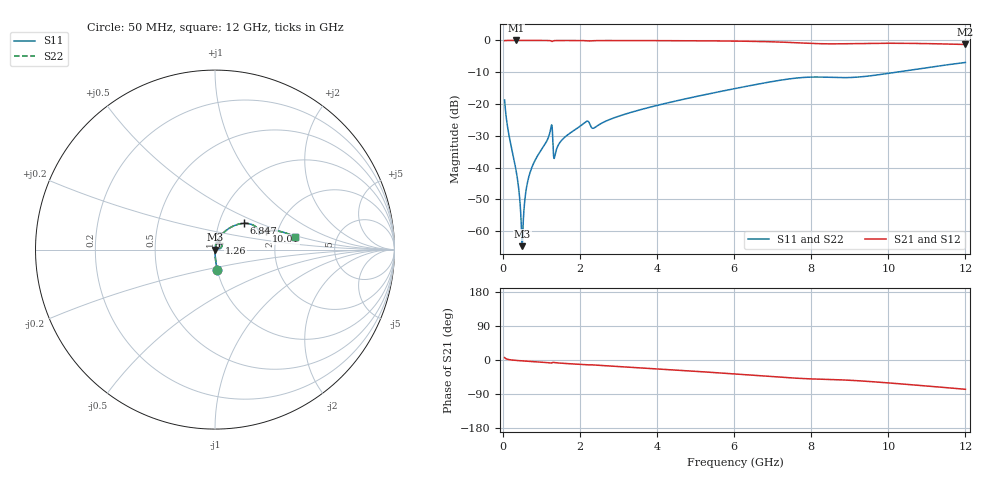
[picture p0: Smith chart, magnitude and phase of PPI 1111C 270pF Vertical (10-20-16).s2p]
# GHz S MA R 50
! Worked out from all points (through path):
!   1601 points, 50 MHz to 12 GHz, reference 50 ohm
!   highest |S21| = 0.00 dB at 348.8 MHz (marker M1); lowest = -1.3 dB at 12 GHz (marker M2)
!   group delay of S21, straight-line fit = 17.6 ps
!   lowest |S11| = -64.7 dB at 505.6 MHz (marker M3), VSWR 1.00, Z = 50.1 - j0.00241 ohm
!   |S11| at or under -10 dB: start of sweep to 10.2 GHz
!   |S22| runs from -64.7 to -6.9 dB; largest |S21 - S12| = 0
!   S11 on the Smith chart (normalised r, x): 50 MHz: 1.00, -0.23; 1.26 GHz: 1.05, +0.08; 6.847 GHz: 1.31, +0.40; 10.01 GHz: 1.74, +0.40; 12 GHz: 2.54, +0.45
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0.05  0.1158 -83.5  0.993 6.4  0.993 6.4  0.1158 -83.5
0.1620312  0.03261 -88.2  0.9991 1.1  0.9991 1.1  0.03261 -88.2
0.34875  0.008913 -87.9  0.9994 -1.1  0.9994 -1.1  0.008913 -87.9
0.4085  0.005073 -85.6  0.9994 -1.6  0.9994 -1.6  0.005073 -85.6
0.46825  0.001894 -74.8  0.9994 -2.0  0.9994 -2.0  0.001894 -74.8
0.5055937  0.000579 -2.4  0.9994 -2.3  0.9994 -2.3  0.000579 -2.4
0.5429375  0.001789 67.9  0.9994 -2.6  0.9994 -2.6  0.001789 67.9
0.6325625  0.005421 80.0  0.9993 -3.2  0.9993 -3.2  0.005421 80.0
0.7296563  0.00906 81.8  0.9992 -3.8  0.9992 -3.8  0.00906 81.8
1.222594  0.0352 73.2  0.9937 -7.6  0.9937 -7.6  0.0352 73.2
1.259937  0.04517 56.5  0.9797 -8.1  0.9797 -8.1  0.04517 56.5
1.371969  0.0172 69.5  0.9958 -7.2  0.9958 -7.2  0.0172 69.5
1.558688  0.02804 78.3  0.9981 -8.7  0.9981 -8.7  0.02804 78.3
2.044156  0.04645 74.2  0.9957 -11.9  0.9957 -11.9  0.04645 74.2
2.193531  0.05377 64.0  0.9864 -13.0  0.9864 -13.0  0.05377 64.0
2.372781  0.04202 66.3  0.9913 -13.1  0.9913 -13.1  0.04202 66.3
4.038312  0.0961 65.0  0.993 -23.7  0.993 -23.7  0.0961 65.0
6.025  0.1749 50.6  0.9764 -36.9  0.9764 -36.9  0.1749 50.6
6.846563  0.2176 42.2  0.9569 -42.8  0.9569 -42.8  0.2176 42.2
8.019156  0.2653 25.0  0.8975 -50.0  0.8975 -50.0  0.2653 25.0
10.01331  0.3041 19.9  0.9029 -60.5  0.9029 -60.5  0.3041 19.9
12  0.4503 9.0  0.8634 -77.3  0.8634 -77.3  0.4503 9.0
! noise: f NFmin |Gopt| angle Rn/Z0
0.05  0.0003431  0.8555  0.3095  0.0005074
1.372  0.007134  0.8141  6.224  0.00799
2.701  0.007703  0.6869  12.02  0.004727
4.031  0.009194  0.6268  17.54  0.004512
5.36  0.015  0.6888  23.35  0.009001
6.682  0.0311  0.8038  29.28  0.03084
8.012  0.07255  0.8962  34.98  0.1389
9.341  0.07722  0.8894  40.3  0.1339
10.67  0.06249  0.8512  45.29  0.07631
12  0.05719  0.825  50.01  0.05653
